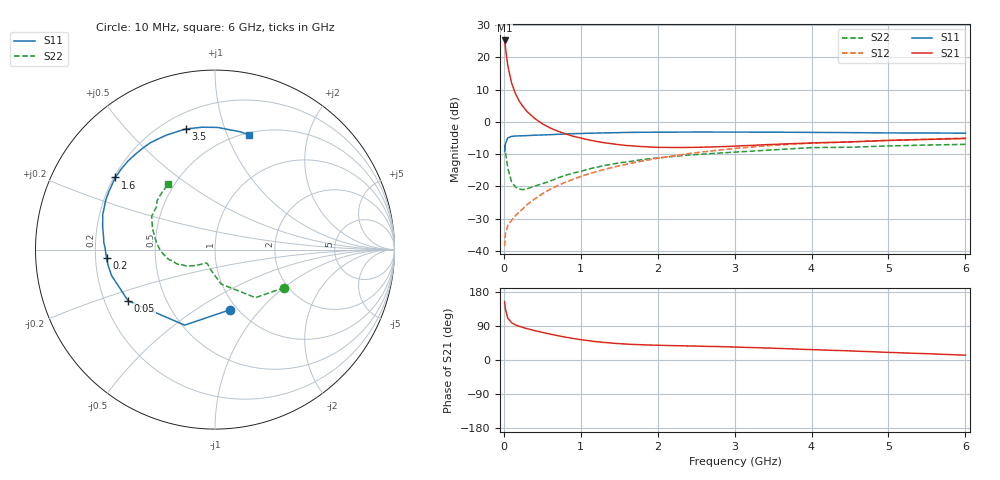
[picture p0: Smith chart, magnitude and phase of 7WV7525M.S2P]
! Infineon Technologies  Discrete & RF Semiconductors
! BFS17W
! Si NPN RF Bipolar Junction Transistor in SOT323
! VCE = 0.75 V  IC = 25 mA
! Common Emitter S-Parameters:  August  1999
# GHz  S  MA  R  50
!  f  S11  S21  S12  S22
! GHz  MAG  ANG  MAG  ANG  MAG  ANG  MAG  ANG
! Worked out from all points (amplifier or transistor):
!   36 points, 10 MHz to 6 GHz, reference 50 ohm
!   highest |S21| = 25.2 dB at 10 MHz (marker M1)
!   |S21| within 3 dB of that: start of sweep to 25.14 MHz
!   unconditionally stable (mu >= 1): start of sweep to end of sweep
!   at 250 MHz: K = 4.05, MAG = 6.8 dB, |S12| = -26.9 dB
!   at 1.4 GHz: K = 3.01, MAG = -4.0 dB, |S12| = -14.2 dB
!   at 6 GHz: K = 1.17, MAG = -2.6 dB, |S12| = -5.0 dB
!   S11 on the Smith chart (normalised r, x): 10 MHz: 0.92, -0.70; 50 MHz: 0.30, -0.25; 200 MHz: 0.25, -0.04; 1.6 GHz: 0.21, +0.31; 3.5 GHz: 0.29, +0.74; 6 GHz: 0.52, +1.20
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0.01  0.3457 -76.2  18.27 153.9  0.0118 61.6  0.4403 -28.7
0.02  0.4536 -111.9  14.44 135.1  0.0181 48.8  0.35 -49.9
0.05  0.562 -149.5  7.587 110.8  0.0246 37.2  0.1949 -79.9
0.1  0.5938 -165.8  4.025 98.5  0.0296 38.5  0.1179 -100.7
0.15  0.6028 -171.9  2.75 92.8  0.0351 45.0  0.0979 -111.3
0.2  0.6054 -175.5  2.098 88.9  0.0399 50.5  0.0904 -116.9
0.25  0.6088 -178.3  1.716 85.8  0.0452 53.9  0.0889 -122.4
0.3  0.6113 179.7  1.45 82.9  0.0517 57.3  0.0915 -124.6
0.4  0.6207 176.3  1.129 77.6  0.0635 61.3  0.1006 -130.6
0.5  0.6253 173.3  0.936 73.0  0.0765 63.9  0.1098 -132.4
0.6  0.6323 170.6  0.804 68.4  0.0895 65.1  0.1204 -135.8
0.7  0.6407 167.8  0.718 64.2  0.1028 66.0  0.1345 -139.6
0.9  0.6557 162.6  0.598 56.9  0.1283 66.1  0.1605 -145.8
1.1  0.6656 156.9  0.525 51.0  0.1556 65.5  0.1849 -150.6
1.3  0.6739 151.3  0.475 46.4  0.182 64.1  0.2091 -156.6
1.6  0.6852 144.1  0.429 41.9  0.2205 61.6  0.239 -163.6
2.2  0.692 130.1  0.4 37.9  0.2968 55.3  0.2902 -175.3
2.8  0.6932 117.1  0.411 35.3  0.3646 47.9  0.3279 173.0
3.5  0.6919 103.7  0.447 31.1  0.4333 39.0  0.3676 161.3
4.5  0.6807 88.6  0.488 24.0  0.4876 27.5  0.4033 144.3
5.5  0.6715 78.0  0.533 16.6  0.5373 18.7  0.4363 132.0
6  0.6667 73.7  0.55 12.7  0.5605 14.3  0.4476 125.4
